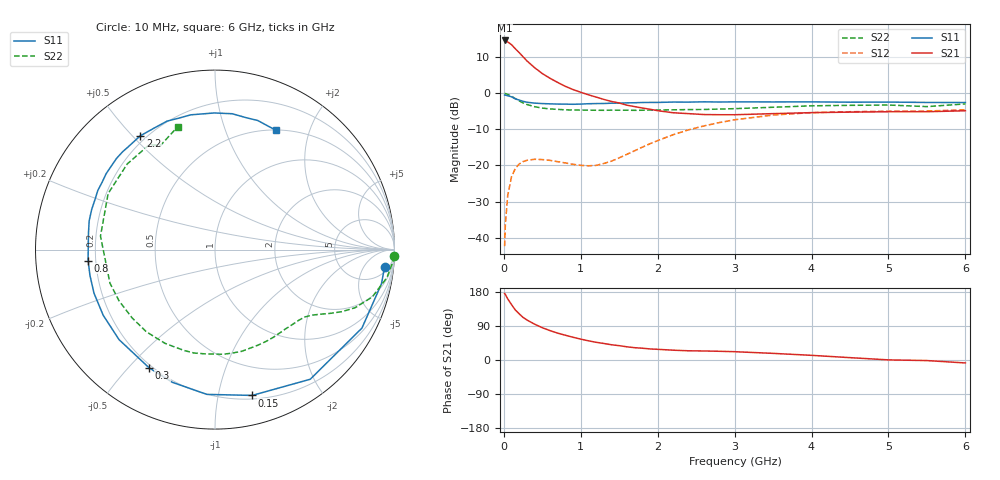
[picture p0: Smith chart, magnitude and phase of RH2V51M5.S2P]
! SIEMENS Small Signal Semiconductors
! BFR106
! Si NPN RF Bipolar Junction Transistor in SOT23
! VCE = 2.5 V  IC = 1.5 mA
! Common Emitter S-Parameters:  August  1996
# GHz  S  MA  R  50
!  f  S11  S21  S12  S22
! GHz  MAG  ANG  MAG  ANG  MAG  ANG  MAG  ANG
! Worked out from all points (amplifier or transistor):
!   36 points, 10 MHz to 6 GHz, reference 50 ohm
!   highest |S21| = 14.7 dB at 10 MHz (marker M1)
!   |S21| within 3 dB of that: start of sweep to 182 MHz
!   unconditionally stable (mu >= 1): 805.2 MHz to 2.166 GHz; 2.682 GHz to end of sweep
!   at 250 MHz: K = 0.29, MSG = 14.5 dB, |S12| = -18.9 dB
!   at 1.4 GHz: K = 1.35, MAG = 4.7 dB, |S12| = -18.8 dB
!   at 6 GHz: K = 1.02, MAG = -1.0 dB, |S12| = -4.6 dB
!   S11 on the Smith chart (normalised r, x): 10 MHz: 8, -16; 150 MHz: 0.23, -1.26; 300 MHz: 0.19, -0.57; 800 MHz: 0.17, -0.04; 2.2 GHz: 0.18, +0.53; 6 GHz: 0.50, +1.51
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0.01  0.9498 -5.8  5.425 175.7  0.0076 87.5  0.9989 -2.1
0.02  0.9469 -11.6  5.385 172.7  0.0152 84.6  0.9937 -3.8
0.05  0.9282 -28.1  5.169 161.4  0.0381 74.0  0.9709 -9.2
0.1  0.8963 -53.7  4.743 146.1  0.0698 61.1  0.9148 -16.8
0.15  0.8384 -75.7  4.153 131.8  0.0913 49.1  0.8455 -22.5
0.2  0.8079 -93.2  3.675 121.7  0.105 41.6  0.788 -26.0
0.25  0.7767 -107.8  3.219 112.4  0.1133 34.8  0.7365 -28.8
0.3  0.7542 -119.1  2.827 105.6  0.118 30.5  0.7021 -30.7
0.4  0.7331 -136.8  2.274 94.5  0.122 24.1  0.654 -33.9
0.5  0.7224 -149.6  1.886 85.2  0.1207 20.4  0.6252 -36.9
0.6  0.7166 -160.2  1.62 77.6  0.1178 18.9  0.6096 -40.4
0.8  0.7097 -175.0  1.252 65.3  0.1084 20.5  0.5916 -48.1
1.1  0.7192 167.1  0.956 50.6  0.0989 34.4  0.5851 -61.1
1.6  0.7395 145.1  0.686 34.8  0.1428 63.0  0.5848 -85.5
2.2  0.7584 123.3  0.539 25.9  0.267 64.5  0.5919 -117.9
2.8  0.7596 105.2  0.506 23.0  0.3935 51.6  0.6062 -151.9
3.5  0.7613 90.3  0.524 17.5  0.5012 34.5  0.6424 173.3
4  0.763 82.8  0.541 12.3  0.5408 23.1  0.6724 152.3
4.5  0.7552 76.8  0.55 6.2  0.5571 13.5  0.6831 135.7
5  0.7577 71.7  0.557 0.3  0.5656 5.7  0.6898 122.1
5.5  0.7489 66.7  0.557 -1.5  0.5699 2.1  0.6556 117.5
6  0.7469 63.1  0.574 -7.8  0.5916 -5.5  0.7151 106.9
